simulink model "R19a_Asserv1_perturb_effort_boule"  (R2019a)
settings: Solver=ode15s  StartTime=0.0  StopTime=1  RelTol=1e-3  EnableMultiTasking=on
undefined symbols (not defined in the file): deg, kg, m, manette1_Défaut_sldprt, manette2_Défaut_sldprt, mm, N, rad, s, sigbuilder_block, STL, X, Y, Z
libraries: sm_lib x460, fl_lib x45, nesl_utility x23, simulink x3
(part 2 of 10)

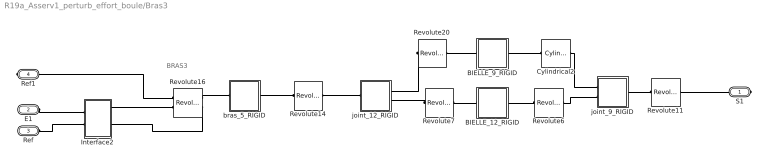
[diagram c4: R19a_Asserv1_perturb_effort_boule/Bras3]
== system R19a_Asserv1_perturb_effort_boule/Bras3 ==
  note: BRAS3
  BIELLE_12_RIGID : Subsystem
  BIELLE_9_RIGID : Subsystem
  Cylindrical2 : sm_lib/Joints/Cylindrical Joint  SenseConstraintForce=off  SenseConstraintForceX=off  SenseConstraintForceY=off  SenseConstraintForceZ=off  SenseConstraintTorque=off  SenseConstraintTorqueX=off  SenseConstraintTorqueY=off  SenseConstraintTorqueZ=off  SenseTotalForce=off  SenseTotalForceX=off  SenseTotalForceY=off  SenseTotalForceZ=off  SenseTotalTorque=off  SenseTotalTorqueX=off  SenseTotalTorqueY=off  SenseTotalTorqueZ=off  CompositeWrenchDir=FollowerOnBase  CompositeWrenchFrame=BaseFrame  PzEquilibriumPosition=0  PzEquilibriumPositionUnits=m  PzSpringStiffness=0  PzSpringStiffnessUnits=N/m  PzDampingCoefficient=0  PzDampingCoefficientUnits=s*N/m  PzTorqueActuationMode=NoTorque  PzMotionActuationMode=ComputedMotion  PzSensePosition=off  PzSenseVelocity=off  PzSenseAcceleration=off  PzSenseTorqueForce=off  PzSenseLowerLimitTorqueForce=off  PzSenseUpperLimitTorqueForce=off  PzLowerLimitSpecify=off  PzLowerLimitBound=-1  PzLowerLimitBoundUnits=m  PzLowerLimitStiffness=1e6  PzLowerLimitStiffnessUnits=N/m  PzLowerLimitDamping=1e3  PzLowerLimitDampingUnits=N/(m/s)  PzLowerLimitTransitionRegionWidth=1e-4  PzLowerLimitTransitionRegionWidthUnits=m  PzUpperLimitSpecify=off  PzUpperLimitBound=1  PzUpperLimitBoundUnits=m  PzUpperLimitStiffness=1e6  PzUpperLimitStiffnessUnits=N/m  PzUpperLimitDamping=1e3  PzUpperLimitDampingUnits=N/(m/s)  PzUpperLimitTransitionRegionWidth=1e-4  PzUpperLimitTransitionRegionWidthUnits=m  PzPositionTargetSpecify=off  PzPositionTargetPriority=High  PzPositionTargetValue=0  PzPositionTargetValueUnits=m  PzVelocityTargetSpecify=off  PzVelocityTargetPriority=High  PzVelocityTargetValue=0  PzVelocityTargetValueUnits=m/s  RzEquilibriumPosition=0  RzEquilibriumPositionUnits=rad  RzSpringStiffness=0  RzSpringStiffnessUnits=m*N/rad  RzDampingCoefficient=0  RzDampingCoefficientUnits=m*s*N/rad  RzTorqueActuationMode=NoTorque  RzMotionActuationMode=ComputedMotion  RzSensePosition=off  RzSenseVelocity=off  RzSenseAcceleration=off  RzSenseTorqueForce=off  RzSenseLowerLimitTorqueForce=off  RzSenseUpperLimitTorqueForce=off  RzLowerLimitSpecify=off  RzLowerLimitBound=-90  RzLowerLimitBoundUnits=deg  RzLowerLimitStiffness=1e4  RzLowerLimitStiffnessUnits=N*m/deg  RzLowerLimitDamping=10  RzLowerLimitDampingUnits=N*m/(deg/s)  RzLowerLimitTransitionRegionWidth=0.1  RzLowerLimitTransitionRegionWidthUnits=deg  RzUpperLimitSpecify=off  RzUpperLimitBound=90  RzUpperLimitBoundUnits=deg  RzUpperLimitStiffness=1e4  RzUpperLimitStiffnessUnits=N*m/deg  RzUpperLimitDamping=10  RzUpperLimitDampingUnits=N*m/(deg/s)  RzUpperLimitTransitionRegionWidth=0.1  RzUpperLimitTransitionRegionWidthUnits=deg  RzPositionTargetSpecify=off  RzPositionTargetPriority=High  RzPositionTargetValue=0  RzPositionTargetValueUnits=deg  RzVelocityTargetSpecify=off  RzVelocityTargetPriority=High  RzVelocityTargetValue=0  RzVelocityTargetValueUnits=deg/s
  Interface2 : Subsystem
  Revolute11 : sm_lib/Joints/Revolute Joint  SenseConstraintForce=off  SenseConstraintForceX=off  SenseConstraintForceY=off  SenseConstraintForceZ=off  SenseConstraintTorque=off  SenseConstraintTorqueX=off  SenseConstraintTorqueY=off  SenseConstraintTorqueZ=off  SenseTotalForce=off  SenseTotalForceX=off  SenseTotalForceY=off  SenseTotalForceZ=off  SenseTotalTorque=off  SenseTotalTorqueX=off  SenseTotalTorqueY=off  SenseTotalTorqueZ=off  CompositeWrenchDir=FollowerOnBase  CompositeWrenchFrame=BaseFrame  EquilibriumPosition=0  EquilibriumPositionUnits=rad  SpringStiffness=0  SpringStiffnessUnits=m*N/rad  DampingCoefficient=0  DampingCoefficientUnits=m*s*N/rad  TorqueActuationMode=NoTorque  MotionActuationMode=ComputedMotion  SensePosition=off  SenseVelocity=off  SenseAcceleration=off  SenseTorqueForce=off  SenseLowerLimitTorqueForce=off  SenseUpperLimitTorqueForce=off  LowerLimitSpecify=off  LowerLimitBound=-90  LowerLimitBoundUnits=deg  LowerLimitStiffness=1e4  LowerLimitStiffnessUnits=N*m/deg  LowerLimitDamping=10  LowerLimitDampingUnits=N*m/(deg/s)  LowerLimitTransitionRegionWidth=0.1  LowerLimitTransitionRegionWidthUnits=deg  UpperLimitSpecify=off  UpperLimitBound=90  UpperLimitBoundUnits=deg  UpperLimitStiffness=1e4  UpperLimitStiffnessUnits=N*m/deg  UpperLimitDamping=10  UpperLimitDampingUnits=N*m/(deg/s)  UpperLimitTransitionRegionWidth=0.1  UpperLimitTransitionRegionWidthUnits=deg  PositionTargetSpecify=on  PositionTargetPriority=Low  PositionTargetValue=36.757042846011267  PositionTargetValueUnits=deg  VelocityTargetSpecify=off  VelocityTargetPriority=High  VelocityTargetValue=0  VelocityTargetValueUnits=deg/s
  Revolute14 : sm_lib/Joints/Revolute Joint  SenseConstraintForce=off  SenseConstraintForceX=off  SenseConstraintForceY=off  SenseConstraintForceZ=off  SenseConstraintTorque=off  SenseConstraintTorqueX=off  SenseConstraintTorqueY=off  SenseConstraintTorqueZ=off  SenseTotalForce=off  SenseTotalForceX=off  SenseTotalForceY=off  SenseTotalForceZ=off  SenseTotalTorque=off  SenseTotalTorqueX=off  SenseTotalTorqueY=off  SenseTotalTorqueZ=off  CompositeWrenchDir=FollowerOnBase  CompositeWrenchFrame=BaseFrame  EquilibriumPosition=0  EquilibriumPositionUnits=rad  SpringStiffness=0  SpringStiffnessUnits=m*N/rad  DampingCoefficient=0  DampingCoefficientUnits=m*s*N/rad  TorqueActuationMode=NoTorque  MotionActuationMode=ComputedMotion  SensePosition=off  SenseVelocity=off  SenseAcceleration=off  SenseTorqueForce=off  SenseLowerLimitTorqueForce=off  SenseUpperLimitTorqueForce=off  LowerLimitSpecify=off  LowerLimitBound=-90  LowerLimitBoundUnits=deg  LowerLimitStiffness=1e4  LowerLimitStiffnessUnits=N*m/deg  LowerLimitDamping=10  LowerLimitDampingUnits=N*m/(deg/s)  LowerLimitTransitionRegionWidth=0.1  LowerLimitTransitionRegionWidthUnits=deg  UpperLimitSpecify=off  UpperLimitBound=90  UpperLimitBoundUnits=deg  UpperLimitStiffness=1e4  UpperLimitStiffnessUnits=N*m/deg  UpperLimitDamping=10  UpperLimitDampingUnits=N*m/(deg/s)  UpperLimitTransitionRegionWidth=0.1  UpperLimitTransitionRegionWidthUnits=deg  PositionTargetSpecify=on  PositionTargetPriority=Low  PositionTargetValue=114.86123956506862  PositionTargetValueUnits=deg  VelocityTargetSpecify=off  VelocityTargetPriority=High  VelocityTargetValue=0  VelocityTargetValueUnits=deg/s
  Revolute16 : sm_lib/Joints/Revolute Joint  SenseConstraintForce=off  SenseConstraintForceX=off  SenseConstraintForceY=off  SenseConstraintForceZ=off  SenseConstraintTorque=off  SenseConstraintTorqueX=off  SenseConstraintTorqueY=off  SenseConstraintTorqueZ=off  SenseTotalForce=off  SenseTotalForceX=off  SenseTotalForceY=off  SenseTotalForceZ=off  SenseTotalTorque=off  SenseTotalTorqueX=off  SenseTotalTorqueY=off  SenseTotalTorqueZ=off  CompositeWrenchDir=FollowerOnBase  CompositeWrenchFrame=BaseFrame  EquilibriumPosition=0  EquilibriumPositionUnits=rad  SpringStiffness=0  SpringStiffnessUnits=m*N/rad  DampingCoefficient=0  DampingCoefficientUnits=m*s*N/rad  TorqueActuationMode=InputTorque  MotionActuationMode=ComputedMotion  SensePosition=off  SenseVelocity=on  SenseAcceleration=off  SenseTorqueForce=off  SenseLowerLimitTorqueForce=off  SenseUpperLimitTorqueForce=off  LowerLimitSpecify=off  LowerLimitBound=-90  LowerLimitBoundUnits=deg  LowerLimitStiffness=1e4  LowerLimitStiffnessUnits=N*m/deg  LowerLimitDamping=10  LowerLimitDampingUnits=N*m/(deg/s)  LowerLimitTransitionRegionWidth=0.1  LowerLimitTransitionRegionWidthUnits=deg  UpperLimitSpecify=off  UpperLimitBound=90  UpperLimitBoundUnits=deg  UpperLimitStiffness=1e4  UpperLimitStiffnessUnits=N*m/deg  UpperLimitDamping=10  UpperLimitDampingUnits=N*m/(deg/s)  UpperLimitTransitionRegionWidth=0.1  UpperLimitTransitionRegionWidthUnits=deg  PositionTargetSpecify=on  PositionTargetPriority=Low  PositionTargetValue=101.89580328094226  PositionTargetValueUnits=deg  VelocityTargetSpecify=off  VelocityTargetPriority=High  VelocityTargetValue=0  VelocityTargetValueUnits=deg/s
  Revolute20 : sm_lib/Joints/Revolute Joint  SenseConstraintForce=off  SenseConstraintForceX=off  SenseConstraintForceY=off  SenseConstraintForceZ=off  SenseConstraintTorque=off  SenseConstraintTorqueX=off  SenseConstraintTorqueY=off  SenseConstraintTorqueZ=off  SenseTotalForce=off  SenseTotalForceX=off  SenseTotalForceY=off  SenseTotalForceZ=off  SenseTotalTorque=off  SenseTotalTorqueX=off  SenseTotalTorqueY=off  SenseTotalTorqueZ=off  CompositeWrenchDir=FollowerOnBase  CompositeWrenchFrame=BaseFrame  EquilibriumPosition=0  EquilibriumPositionUnits=rad  SpringStiffness=0  SpringStiffnessUnits=m*N/rad  DampingCoefficient=0  DampingCoefficientUnits=m*s*N/rad  TorqueActuationMode=NoTorque  MotionActuationMode=ComputedMotion  SensePosition=off  SenseVelocity=off  SenseAcceleration=off  SenseTorqueForce=off  SenseLowerLimitTorqueForce=off  SenseUpperLimitTorqueForce=off  LowerLimitSpecify=off  LowerLimitBound=-90  LowerLimitBoundUnits=deg  LowerLimitStiffness=1e4  LowerLimitStiffnessUnits=N*m/deg  LowerLimitDamping=10  LowerLimitDampingUnits=N*m/(deg/s)  LowerLimitTransitionRegionWidth=0.1  LowerLimitTransitionRegionWidthUnits=deg  UpperLimitSpecify=off  UpperLimitBound=90  UpperLimitBoundUnits=deg  UpperLimitStiffness=1e4  UpperLimitStiffnessUnits=N*m/deg  UpperLimitDamping=10  UpperLimitDampingUnits=N*m/(deg/s)  UpperLimitTransitionRegionWidth=0.1  UpperLimitTransitionRegionWidthUnits=deg  PositionTargetSpecify=on  PositionTargetPriority=Low  PositionTargetValue=-178.83470303505044  PositionTargetValueUnits=deg  VelocityTargetSpecify=off  VelocityTargetPriority=High  VelocityTargetValue=0  VelocityTargetValueUnits=deg/s
  Revolute6 : sm_lib/Joints/Revolute Joint  SenseConstraintForce=off  SenseConstraintForceX=off  SenseConstraintForceY=off  SenseConstraintForceZ=off  SenseConstraintTorque=off  SenseConstraintTorqueX=off  SenseConstraintTorqueY=off  SenseConstraintTorqueZ=off  SenseTotalForce=off  SenseTotalForceX=off  SenseTotalForceY=off  SenseTotalForceZ=off  SenseTotalTorque=off  SenseTotalTorqueX=off  SenseTotalTorqueY=off  SenseTotalTorqueZ=off  CompositeWrenchDir=FollowerOnBase  CompositeWrenchFrame=BaseFrame  EquilibriumPosition=0  EquilibriumPositionUnits=rad  SpringStiffness=0  SpringStiffnessUnits=m*N/rad  DampingCoefficient=0  DampingCoefficientUnits=m*s*N/rad  TorqueActuationMode=NoTorque  MotionActuationMode=ComputedMotion  SensePosition=off  SenseVelocity=off  SenseAcceleration=off  SenseTorqueForce=off  SenseLowerLimitTorqueForce=off  SenseUpperLimitTorqueForce=off  LowerLimitSpecify=off  LowerLimitBound=-90  LowerLimitBoundUnits=deg  LowerLimitStiffness=1e4  LowerLimitStiffnessUnits=N*m/deg  LowerLimitDamping=10  LowerLimitDampingUnits=N*m/(deg/s)  LowerLimitTransitionRegionWidth=0.1  LowerLimitTransitionRegionWidthUnits=deg  UpperLimitSpecify=off  UpperLimitBound=90  UpperLimitBoundUnits=deg  UpperLimitStiffness=1e4  UpperLimitStiffnessUnits=N*m/deg  UpperLimitDamping=10  UpperLimitDampingUnits=N*m/(deg/s)  UpperLimitTransitionRegionWidth=0.1  UpperLimitTransitionRegionWidthUnits=deg  PositionTargetSpecify=on  PositionTargetPriority=Low  PositionTargetValue=-178.83470303504936  PositionTargetValueUnits=deg  VelocityTargetSpecify=off  VelocityTargetPriority=High  VelocityTargetValue=0  VelocityTargetValueUnits=deg/s
  Revolute7 : sm_lib/Joints/Revolute Joint  SenseConstraintForce=off  SenseConstraintForceX=off  SenseConstraintForceY=off  SenseConstraintForceZ=off  SenseConstraintTorque=off  SenseConstraintTorqueX=off  SenseConstraintTorqueY=off  SenseConstraintTorqueZ=off  SenseTotalForce=off  SenseTotalForceX=off  SenseTotalForceY=off  SenseTotalForceZ=off  SenseTotalTorque=off  SenseTotalTorqueX=off  SenseTotalTorqueY=off  SenseTotalTorqueZ=off  CompositeWrenchDir=FollowerOnBase  CompositeWrenchFrame=BaseFrame  EquilibriumPosition=0  EquilibriumPositionUnits=rad  SpringStiffness=0  SpringStiffnessUnits=m*N/rad  DampingCoefficient=0  DampingCoefficientUnits=m*s*N/rad  TorqueActuationMode=NoTorque  MotionActuationMode=ComputedMotion  SensePosition=off  SenseVelocity=off  SenseAcceleration=off  SenseTorqueForce=off  SenseLowerLimitTorqueForce=off  SenseUpperLimitTorqueForce=off  LowerLimitSpecify=off  LowerLimitBound=-90  LowerLimitBoundUnits=deg  LowerLimitStiffness=1e4  LowerLimitStiffnessUnits=N*m/deg  LowerLimitDamping=10  LowerLimitDampingUnits=N*m/(deg/s)  LowerLimitTransitionRegionWidth=0.1  LowerLimitTransitionRegionWidthUnits=deg  UpperLimitSpecify=off  UpperLimitBound=90  UpperLimitBoundUnits=deg  UpperLimitStiffness=1e4  UpperLimitStiffnessUnits=N*m/deg  UpperLimitDamping=10  UpperLimitDampingUnits=N*m/(deg/s)  UpperLimitTransitionRegionWidth=0.1  UpperLimitTransitionRegionWidthUnits=deg  PositionTargetSpecify=on  PositionTargetPriority=Low  PositionTargetValue=1.1652969649496245  PositionTargetValueUnits=deg  VelocityTargetSpecify=off  VelocityTargetPriority=High  VelocityTargetValue=0  VelocityTargetValueUnits=deg/s
  bras_5_RIGID : Subsystem
  joint_12_RIGID : Subsystem
  joint_9_RIGID : Subsystem
  S1 : PMIOPort  Side=Right
  E1 : PMIOPort  Port=2  Side=Left
  Ref : PMIOPort  Port=3  Side=Left
  Ref1 : PMIOPort  Port=4  Side=Right
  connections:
  Interface2/RConn2 -- Revolute16/RConn2
  Interface2/RConn1 -- Revolute16/LConn2
  E1/RConn1 -- Interface2/LConn1
  Ref/RConn1 -- Interface2/LConn2
  Revolute11/RConn1 -- joint_9_RIGID/RConn1
  Revolute7/RConn1 -- joint_12_RIGID/RConn2
  Revolute14/RConn1 -- joint_12_RIGID/LConn1
  S1/RConn1 -- Revolute11/LConn1
  Revolute14/LConn1 -- bras_5_RIGID/RConn1
  Revolute16/LConn1 -- Ref1/RConn1
  Revolute16/RConn1 -- bras_5_RIGID/LConn1
  BIELLE_12_RIGID/RConn1 -- Revolute6/LConn1
  BIELLE_12_RIGID/LConn1 -- Revolute7/LConn1
  Revolute6/RConn1 -- joint_9_RIGID/LConn2
  Revolute20/RConn1 -- joint_12_RIGID/RConn1
  BIELLE_9_RIGID/LConn1 -- Revolute20/LConn1
  BIELLE_9_RIGID/RConn1 -- Cylindrical2/LConn1
  Cylindrical2/RConn1 -- joint_9_RIGID/LConn1

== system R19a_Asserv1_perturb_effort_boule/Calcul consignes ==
  note: a = 0.06; b = 0.1025; c = 0.014; d = 0.01125; e = 0.01125; f = 0.025 ; r = 0.03723; s = 0.02733;
  In1 : Inport
  In2 : Inport  Port=2
  In3 : Inport  Port=3
  AngleMoteur1 : MATLAB Function  TreatAsAtomicUnit=on
  AngleMoteur2 : MATLAB Function  TreatAsAtomicUnit=on
  AngleMoteur3 : MATLAB Function  TreatAsAtomicUnit=on
  C1 : Outport
  C2 : Outport  Port=2
  C3 : Outport  Port=3
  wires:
  In3/1 -> AngleMoteur1/3(z), AngleMoteur2/3(z), AngleMoteur3/3(z)
  AngleMoteur2/1(anglmot2) -> C2/1  "Consigne2"
  In1/1 -> AngleMoteur1/1(x), AngleMoteur2/1(x), AngleMoteur3/1(x)
  In2/1 -> AngleMoteur1/2(y), AngleMoteur2/2(y), AngleMoteur3/2(y)
  AngleMoteur1/1(anglmot1) -> C1/1  "Consigne1"
  AngleMoteur3/1(anglmot3) -> C3/1  "Consigne3"

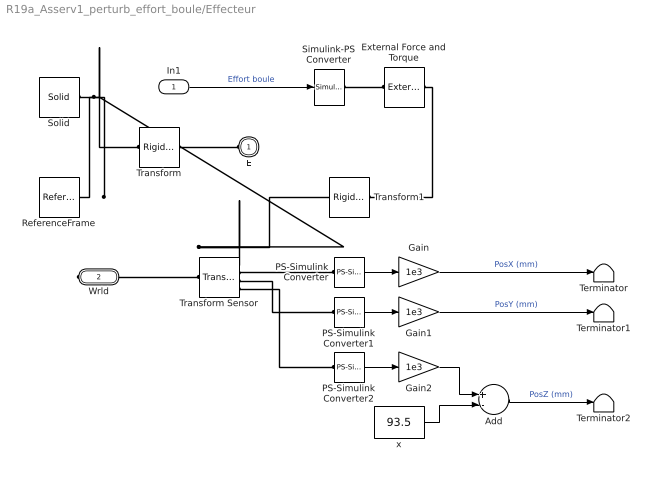
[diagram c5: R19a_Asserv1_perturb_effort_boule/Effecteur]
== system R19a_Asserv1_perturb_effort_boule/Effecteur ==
  In1 : Inport
  Add : Sum  Inputs=+-
  External Force and Torque : sm_lib/Forces and Torques/External Force and Torque  ForceResolutionFrame=AttachedFrame  EnableForceX=off  EnableForceY=off  EnableForceZ=on  EnableForce=off  TorqueResolutionFrame=AttachedFrame  EnableTorqueX=off  EnableTorqueY=off  EnableTorqueZ=off  EnableTorque=off
  Gain : Gain  Gain=1e3
  Gain1 : Gain  Gain=1e3
  Gain2 : Gain  Gain=1e3
  PS-Simulink Converter : nesl_utility/PS-Simulink Converter  PhysicalDomain=network_engine_domain  SubClassName=ps_output  LeftPortType=input  RightPortType=output  PseudoPeriodic=off  Frequencies=[]  Unit=1  AffineConversion=off
  PS-Simulink Converter1 : nesl_utility/PS-Simulink Converter  PhysicalDomain=network_engine_domain  SubClassName=ps_output  LeftPortType=input  RightPortType=output  PseudoPeriodic=off  Frequencies=[]  Unit=1  AffineConversion=off
  PS-Simulink Converter2 : nesl_utility/PS-Simulink Converter  PhysicalDomain=network_engine_domain  SubClassName=ps_output  LeftPortType=input  RightPortType=output  PseudoPeriodic=off  Frequencies=[]  Unit=1  AffineConversion=off
  ReferenceFrame : sm_lib/Frames and Transforms/Reference Frame
  Simulink-PS Converter : nesl_utility/Simulink-PS Converter  PhysicalDomain=network_engine_domain  SubClassName=ps_input  LeftPortType=input  RightPortType=output  PseudoPeriodic=off  Frequencies=[]  NoiseDistribution=none  NoiseParameters=[]  Unit=1  AffineConversion=off  FilteringAndDerivatives=zero  SimscapeFilterOrder=1  InputFilterTimeConstant=0.001  UdotUserProvided=1
  Solid : sm_lib/Body Elements/Solid  InertiaType=Custom  Mass=0.053  MassUnits=kg  CenterOfMass=[0 0 35.7]  CenterOfMassUnits=mm  MomentsOfInertia=[11.53195593564609 11.464562757624146 11.477456236480506]  MomentsOfInertiaUnits=kg*mm^2  ProductsOfInertia=[-0.014032469477280249 0.0038968914795150661 0.025527028661124163]  ProductsOfInertiaUnits=kg*mm^2  BasedOnType=Density  Density=1000  DensityUnits=kg/(m^3)  DoExposeReferenceFrame=on  SerializedFrames=<Frames/>  GraphicType=FromGeometry  MarkerShape=Sphere  MarkerSize=10  MarkerSizeUnits=m  GraphicVisPropType=SimpleVisualProperties  GraphicDiffuseColor=[1 1 1]  GraphicSpecularColor=[0.5 0.5 0.5 1.0]  GraphicAmbientColor=[0.15 0.15 0.15 1.0]  GraphicEmissiveColor=[0.0 0.0 0.0 1.0]  GraphicShininess=75  GraphicOpacity=1  GeometryShape=FromFile  RectangleSize=[1 1]  RectangleSizeUnits=m  BrickDimensions=[1 1 1]  BrickDimensionUnits=m  CylinderRadius=1  CylinderRadiusUnits=m  CylinderLength=1  CylinderLengthUnits=m  SphereRadius=1  SphereRadiusUnits=m  EllipsoidRadii=[1 1 1]  EllipsoidRadiiUnits=m  ExtrusionCrossSection=[1 1; -1 1; -1 -1; 1 -1]  ExtrusionCrossSectionUnits=m  ExtrusionLength=1  ExtrusionLengthUnits=m  PolygonNumSides=3  PolygonOuterRadius=1  PolygonOuterRadiusUnits=m  ExtGeomFileType=STL  ExtGeomFileName=\STL\manette2_Défaut_sldprt.STL  ExtGeomFileUnits=mm  RevolutionCrossSection=[1 1; 1 -1; 2 -1; 2 1]  RevolutionCrossSectionUnits=m  RevolutionExtent=Full  RevolutionAngle=180  RevolutionAngleUnits=deg
  Terminator : Terminator
  Terminator1 : Terminator
  Terminator2 : Terminator
  Transform : sm_lib/Frames and Transforms/Rigid Transform  TranslationMethod=Cartesian  TranslationStandardOffset=0  TranslationLengthUnit=mm  TranslationStandardAxis=+Z  TranslationCartesianOffset=[-0.52204305767083048 1.5422448888264837 -2.2456176397956377e-14]  TranslationROffset=0  TranslationROffsetUnits=m  TranslationZOffset=0  TranslationZOffsetUnits=m  TranslationThetaOffset=0  TranslationThetaOffsetUnits=deg  RotationMethod=ArbitraryAxis  RotationAngleUnits=rad  RotationStandardAxis=+Z  RotationAngle=2.2920311904365782  RotationArbitraryAxis=[0.63063758405056181 -0.45231899713116352 0.63063758405056158]  FollAlignAxisA=+X  BaseAlignAxisA=+Y  FollAlignAxisB=+Y  BaseAlignAxisB=+Z  RotationSequenceAxes=FollowerAxes  RotationSequence=XYX  RotationSequenceAngles=[0 0 0]  RotationSequenceAnglesUnits=deg  RotationMatrix=[1 0 0; 0 1 0; 0 0 1]
  Transform Sensor : sm_lib/Frames and Transforms/Transform Sensor  MeasurementFrame=World  SenseAngle=off  SenseAxis=off  SenseAngle1=off  SenseAngle2=off  SenseAngle3=off  SenseQ=off  SenseR=off  SenseOmegaX=off  SenseOmegaY=off  SenseOmegaZ=off  SenseOmega1=off  SenseOmega2=off  SenseOmega3=off  SenseQDot=off  SenseRDot=off  SenseAlphaX=off  SenseAlphaY=off  SenseAlphaZ=off  SenseAlpha1=off  SenseAlpha2=off  SenseAlpha3=off  SenseQDDot=off  SenseRDDot=off  SenseX=on  SenseY=on  SenseZ=on  SenseRad=off  SenseAzim=off  SenseDist=off  SenseInc=off  SenseXDot=off  SenseYDot=off  SenseZDot=off  SenseRadDot=off  SenseAzimDot=off  SenseDistDot=off  SenseIncDot=off  SenseXDDot=off  SenseYDDot=off  SenseZDDot=off  SenseRadDDot=off  SenseAzimDDot=off  SenseDistDDot=off  SenseIncDDot=off
  Transform1 : sm_lib/Frames and Transforms/Rigid Transform  TranslationMethod=None  TranslationStandardOffset=3  TranslationLengthUnit=mm  TranslationStandardAxis=-Z  TranslationCartesianOffset=[0 0 0]  TranslationROffset=0  TranslationROffsetUnits=m  TranslationZOffset=0  TranslationZOffsetUnits=m  TranslationThetaOffset=0  TranslationThetaOffsetUnits=deg  RotationMethod=None  RotationAngleUnits=rad  RotationStandardAxis=+Z  RotationAngle=2.2920311904365782  RotationArbitraryAxis=[0 0 0]  FollAlignAxisA=+X  BaseAlignAxisA=+Y  FollAlignAxisB=+Y  BaseAlignAxisB=+Z  RotationSequenceAxes=FollowerAxes  RotationSequence=XYX  RotationSequenceAngles=[0 0 0]  RotationSequenceAnglesUnits=deg  RotationMatrix=[1 0 0; 0 1 0; 0 0 1]
  x : Constant  Value=93.5
  E : PMIOPort  Side=Left
  Wrld : PMIOPort  Port=2  Side=Right
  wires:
  Gain1/1 -> Terminator1/1  "PosY (mm)"
  PS-Simulink Converter2/1 -> Gain2/1
  x/1 -> Add/2
  Add/1 -> Terminator2/1  "PosZ (mm)"
  PS-Simulink Converter1/1 -> Gain1/1
  Gain2/1 -> Add/1
  PS-Simulink Converter/1 -> Gain/1
  Gain/1 -> Terminator/1  "PosX (mm)"
  In1/1 -> Simulink-PS Converter/1  "Effort boule"
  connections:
  Solid/RConn1 -- ReferenceFrame/RConn1 -- Transform Sensor/RConn1 -- Transform1/RConn1 -- Transform/LConn1
  Transform/RConn1 -- E/RConn1
  Transform Sensor/RConn3 -- PS-Simulink Converter1/LConn1
  Wrld/RConn1 -- Transform Sensor/LConn1
  PS-Simulink Converter2/LConn1 -- Transform Sensor/RConn4
  Transform Sensor/RConn2 -- PS-Simulink Converter/LConn1
  Simulink-PS Converter/RConn1 -- External Force and Torque/LConn1
  External Force and Torque/RConn1 -- Transform1/LConn1

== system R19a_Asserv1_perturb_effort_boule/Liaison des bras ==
  EFFECTEUR_1_RIGID : Subsystem
  manette_1_RIGID : Subsystem
  E1 : PMIOPort  Side=Left
  E2 : PMIOPort  Port=2  Side=Left
  S1 : PMIOPort  Port=3  Side=Right
  E3 : PMIOPort  Port=4  Side=Left
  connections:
  EFFECTEUR_1_RIGID/RConn1 -- manette_1_RIGID/LConn1
  S1/RConn1 -- manette_1_RIGID/RConn1
  EFFECTEUR_1_RIGID/LConn1 -- E2/RConn1
  EFFECTEUR_1_RIGID/LConn3 -- E1/RConn1
  EFFECTEUR_1_RIGID/LConn2 -- E3/RConn1

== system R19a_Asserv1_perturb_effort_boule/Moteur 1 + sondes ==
  In1 : Inport
  Moteur à courant continu1 : Subsystem
  Reference electrique : fl_lib/Electrical/Electrical Elements/Electrical Reference
  Simulink-PS Converter1 : nesl_utility/Simulink-PS Converter  PhysicalDomain=network_engine_domain  SubClassName=ps_input  LeftPortType=input  RightPortType=output  PseudoPeriodic=off  Frequencies=[]  NoiseDistribution=none  NoiseParameters=[]  Unit=V  AffineConversion=off  FilteringAndDerivatives=zero  SimscapeFilterOrder=2  InputFilterTimeConstant=1e-4  UdotUserProvided=1
  Sondes électriques1 : Subsystem
  Source de tension controlée1 : fl_lib/Electrical/Electrical Sources/Controlled Voltage Source
  Conn1 : PMIOPort  Side=Right
  Conn2 : PMIOPort  Port=2  Side=Right
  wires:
  In1/1 -> Simulink-PS Converter1/1
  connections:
  Conn2/RConn1 -- Moteur à courant continu1/RConn2
  Conn1/RConn1 -- Moteur à courant continu1/RConn1
  Source de tension controlée1/LConn1 -- Sondes électriques1/LConn1
  Simulink-PS Converter1/RConn1 -- Source de tension controlée1/RConn1
  Sondes électriques1/RConn2 -- Source de tension controlée1/RConn2 -- Reference electrique/LConn1 -- Moteur à courant continu1/LConn2
  Sondes électriques1/RConn1 -- Moteur à courant continu1/LConn1

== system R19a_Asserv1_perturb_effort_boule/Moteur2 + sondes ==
  In1 : Inport
  Moteur à courant continu2 : Subsystem
  Reference electrique : fl_lib/Electrical/Electrical Elements/Electrical Reference
  Simulink-PS Converter1 : nesl_utility/Simulink-PS Converter  PhysicalDomain=network_engine_domain  SubClassName=ps_input  LeftPortType=input  RightPortType=output  PseudoPeriodic=off  Frequencies=[]  NoiseDistribution=none  NoiseParameters=[]  Unit=V  AffineConversion=off  FilteringAndDerivatives=zero  SimscapeFilterOrder=2  InputFilterTimeConstant=1e-4  UdotUserProvided=1
  Sondes électriques : Subsystem
  Source de tension controlée : fl_lib/Electrical/Electrical Sources/Controlled Voltage Source
  Conn1 : PMIOPort  Side=Right
  Conn2 : PMIOPort  Port=2  Side=Right
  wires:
  In1/1 -> Simulink-PS Converter1/1
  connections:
  Sondes électriques/RConn1 -- Moteur à courant continu2/LConn1
  Source de tension controlée/RConn2 -- Reference electrique/LConn1 -- Sondes électriques/RConn2 -- Moteur à courant continu2/LConn2
  Simulink-PS Converter1/RConn1 -- Source de tension controlée/RConn1
  Source de tension controlée/LConn1 -- Sondes électriques/LConn1
  Conn1/RConn1 -- Moteur à courant continu2/RConn1
  Conn2/RConn1 -- Moteur à courant continu2/RConn2

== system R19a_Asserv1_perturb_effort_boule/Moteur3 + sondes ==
  In1 : Inport
  Moteur à courant continu3 : Subsystem
  Reference electrique : fl_lib/Electrical/Electrical Elements/Electrical Reference
  Simulink-PS Converter1 : nesl_utility/Simulink-PS Converter  PhysicalDomain=network_engine_domain  SubClassName=ps_input  LeftPortType=input  RightPortType=output  PseudoPeriodic=off  Frequencies=[]  NoiseDistribution=none  NoiseParameters=[]  Unit=V  AffineConversion=off  FilteringAndDerivatives=zero  SimscapeFilterOrder=2  InputFilterTimeConstant=1e-4  UdotUserProvided=1
  Sondes électriques3 : Subsystem
  Source de tension controlée3 : fl_lib/Electrical/Electrical Sources/Controlled Voltage Source
  Conn1 : PMIOPort  Side=Right
  Conn2 : PMIOPort  Port=2  Side=Right
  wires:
  In1/1 -> Simulink-PS Converter1/1
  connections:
  Sondes électriques3/RConn1 -- Moteur à courant continu3/LConn1
  Moteur à courant continu3/LConn2 -- Reference electrique/LConn1 -- Source de tension controlée3/RConn2 -- Sondes électriques3/RConn2
  Simulink-PS Converter1/RConn1 -- Source de tension controlée3/RConn1
  Source de tension controlée3/LConn1 -- Sondes électriques3/LConn1
  Conn1/RConn1 -- Moteur à courant continu3/RConn1
  Conn2/RConn1 -- Moteur à courant continu3/RConn2

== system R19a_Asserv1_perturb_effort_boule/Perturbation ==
  Générateur de perturbation : Subsystem  Tag=STV Subsys  LoadFcn=sigbuilder_block('load');  StartFcn=sigbuilder_block('start');  StopFcn=sigbuilder_block('stop');  ClipboardFcn=sigbuilder_block('clipboard');  mask(Sigbuilder block){tuvar=[0:10]}
      mask help: Simulink:masks:SigbuilderBlock_MD
      mask init:
      | if ~strcmp(get_param(bdroot(gcbh),'SimulationStatus'),'stopped') tuvar = sigbuilder_block('maskInit'); end
  Nul : Constant  Value=0
  Out1 : Outport
  Out2 : Outport  Port=2
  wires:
  Générateur de perturbation/1(Signal 1) -> Out1/1  "On"
  Nul/1 -> Out2/1  "Off"

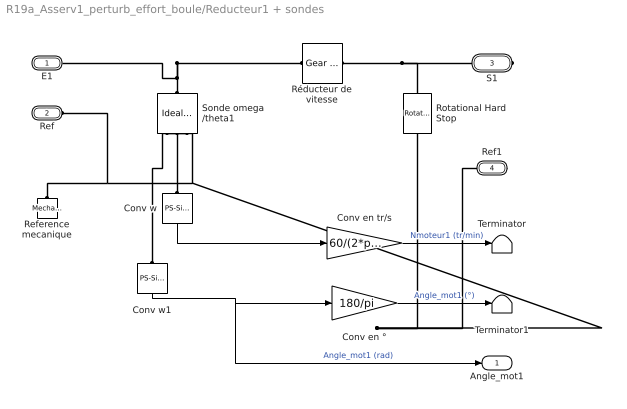
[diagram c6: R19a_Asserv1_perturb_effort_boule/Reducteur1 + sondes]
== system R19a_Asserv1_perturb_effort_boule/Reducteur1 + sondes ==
  Conv en tr/s : Gain  Gain=60/(2*pi)
  Conv en ° : Gain  Gain=180/pi
  Conv w : nesl_utility/PS-Simulink Converter  PhysicalDomain=network_engine_domain  SubClassName=ps_output  LeftPortType=input  RightPortType=output  PseudoPeriodic=off  Frequencies=[]  Unit=1  AffineConversion=off
  Conv w1 : nesl_utility/PS-Simulink Converter  PhysicalDomain=network_engine_domain  SubClassName=ps_output  LeftPortType=input  RightPortType=output  PseudoPeriodic=off  Frequencies=[]  Unit=1  AffineConversion=off
  Reference mecanique : fl_lib/Mechanical/Rotational Elements/Mechanical Rotational Reference
  Rotational Hard Stop : fl_lib/Mechanical/Rotational Elements/Rotational Hard Stop  upper_bnd=0 rad  lower_bnd=-2 rad  stiff_up=1e2 N*m/rad  stiff_low=1e2 N*m/rad  D_up=0.01 N*m/(rad/s)  D_low=0.01 N*m/(rad/s)  model=simscape.enum.hardstop.fulldamped  transition=0.001 rad  w_specify=off  w_priority=High  w=0 rad/s  w_nominal_specify=off  w_nominal_unit=rad/s  w_nominal_value=1  t_specify=off  t_priority=High  t=0 N*m  t_nominal_specify=off  t_nominal_unit=N*m  t_nominal_value=1  phi_specify=off  phi_priority=High  phi=0 rad  phi_nominal_specify=off  phi_nominal_unit=rad  phi_nominal_value=1
  Réducteur de vitesse : fl_lib/Mechanical/Mechanisms/Gear Box  ratio=-7.627  t_in_specify=off  t_in_priority=High  t_in=0 N*m  t_in_nominal_specify=off  t_in_nominal_unit=N*m  t_in_nominal_value=1  t_out_specify=off  t_out_priority=High  t_out=0 N*m  t_out_nominal_specify=off  t_out_nominal_unit=N*m  t_out_nominal_value=1
  Sonde omega /theta1 : fl_lib/Mechanical/Mechanical Sensors/Ideal Rotational Motion Sensor  offset=0 rad
  Terminator : Terminator
  Terminator1 : Terminator
  E1 : PMIOPort  Side=Left
  Ref : PMIOPort  Port=2  Side=Left
  S1 : PMIOPort  Port=3  Side=Right
  Ref1 : PMIOPort  Port=4  Side=Right
  Angle_mot1 : Outport
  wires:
  Conv w1/1 -> Angle_mot1/1, Conv en °/1  "Angle_mot1 (rad)"
  Conv en °/1 -> Terminator1/1  "Angle_mot1 (°)"
  Conv w/1 -> Conv en tr/s/1
  Conv en tr/s/1 -> Terminator/1  "Nmoteur1 (tr/min)"
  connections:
  Sonde omega /theta1/LConn1 -- E1/RConn1 -- Réducteur de vitesse/LConn1
  Reference mecanique/LConn1 -- Ref/RConn1 -- Rotational Hard Stop/RConn1 -- Ref1/RConn1 -- Sonde omega /theta1/RConn1
  Conv w/LConn1 -- Sonde omega /theta1/RConn2
  Conv w1/LConn1 -- Sonde omega /theta1/RConn3
  Réducteur de vitesse/RConn1 -- Rotational Hard Stop/LConn1 -- S1/RConn1

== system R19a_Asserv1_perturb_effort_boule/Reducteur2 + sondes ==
  Conv en tr/s : Gain  Gain=60/(2*pi)
  Conv en ° : Gain  Gain=180/pi
  Conv w : nesl_utility/PS-Simulink Converter  PhysicalDomain=network_engine_domain  SubClassName=ps_output  LeftPortType=input  RightPortType=output  PseudoPeriodic=off  Frequencies=[]  Unit=1  AffineConversion=off
  Conv w1 : nesl_utility/PS-Simulink Converter  PhysicalDomain=network_engine_domain  SubClassName=ps_output  LeftPortType=input  RightPortType=output  PseudoPeriodic=off  Frequencies=[]  Unit=1  AffineConversion=off
  Reference mecanique : fl_lib/Mechanical/Rotational Elements/Mechanical Rotational Reference
  Rotational Hard Stop : fl_lib/Mechanical/Rotational Elements/Rotational Hard Stop  upper_bnd=2 rad  lower_bnd=0 rad  stiff_up=1e2 N*m/rad  stiff_low=1e2 N*m/rad  D_up=0.01 N*m/(rad/s)  D_low=0.01 N*m/(rad/s)  model=simscape.enum.hardstop.fulldamped  transition=0.001 rad  w_specify=off  w_priority=High  w=0 rad/s  w_nominal_specify=off  w_nominal_unit=rad/s  w_nominal_value=1  t_specify=off  t_priority=High  t=0 N*m  t_nominal_specify=off  t_nominal_unit=N*m  t_nominal_value=1  phi_specify=off  phi_priority=High  phi=0 rad  phi_nominal_specify=off  phi_nominal_unit=rad  phi_nominal_value=1
  Réducteur de vitesse2 : fl_lib/Mechanical/Mechanisms/Gear Box  ratio=7.627  t_in_specify=off  t_in_priority=High  t_in=0 N*m  t_in_nominal_specify=off  t_in_nominal_unit=N*m  t_in_nominal_value=1  t_out_specify=off  t_out_priority=High  t_out=0 N*m  t_out_nominal_specify=off  t_out_nominal_unit=N*m  t_out_nominal_value=1
  Sonde omega /theta2 : fl_lib/Mechanical/Mechanical Sensors/Ideal Rotational Motion Sensor  offset=0 rad
  Terminator : Terminator
  Terminator1 : Terminator
  E1 : PMIOPort  Side=Left
  Ref : PMIOPort  Port=2  Side=Left
  S1 : PMIOPort  Port=3  Side=Right
  Ref1 : PMIOPort  Port=4  Side=Right
  Angle_mot2 : Outport
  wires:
  Conv w1/1 -> Angle_mot2/1, Conv en °/1  "Angle_mot2 (rad)"
  Conv en °/1 -> Terminator1/1  "Angle_mot2 (°)"
  Conv w/1 -> Conv en tr/s/1
  Conv en tr/s/1 -> Terminator/1  "Nmoteur2 (tr/min)"
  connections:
  Sonde omega /theta2/LConn1 -- E1/RConn1 -- Réducteur de vitesse2/LConn1
  Ref1/RConn1 -- Rotational Hard Stop/RConn1 -- Sonde omega /theta2/RConn1 -- Reference mecanique/LConn1 -- Ref/RConn1
  Conv w1/LConn1 -- Sonde omega /theta2/RConn3
  Conv w/LConn1 -- Sonde omega /theta2/RConn2
  Réducteur de vitesse2/RConn1 -- Rotational Hard Stop/LConn1 -- S1/RConn1

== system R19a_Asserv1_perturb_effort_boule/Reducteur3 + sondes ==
  Conv en tr/s : Gain  Gain=60/(2*pi)
  Conv en ° : Gain  Gain=180/pi
  Conv w : nesl_utility/PS-Simulink Converter  PhysicalDomain=network_engine_domain  SubClassName=ps_output  LeftPortType=input  RightPortType=output  PseudoPeriodic=off  Frequencies=[]  Unit=1  AffineConversion=off
  Conv w1 : nesl_utility/PS-Simulink Converter  PhysicalDomain=network_engine_domain  SubClassName=ps_output  LeftPortType=input  RightPortType=output  PseudoPeriodic=off  Frequencies=[]  Unit=1  AffineConversion=off
  Reference mecanique : fl_lib/Mechanical/Rotational Elements/Mechanical Rotational Reference
  Rotational Hard Stop : fl_lib/Mechanical/Rotational Elements/Rotational Hard Stop  upper_bnd=2 rad  lower_bnd=0 rad  stiff_up=1e2 N*m/rad  stiff_low=1e2 N*m/rad  D_up=0.01 N*m/(rad/s)  D_low=0.01 N*m/(rad/s)  model=simscape.enum.hardstop.fulldamped  transition=0.001 rad  w_specify=off  w_priority=High  w=0 rad/s  w_nominal_specify=off  w_nominal_unit=rad/s  w_nominal_value=1  t_specify=off  t_priority=High  t=0 N*m  t_nominal_specify=off  t_nominal_unit=N*m  t_nominal_value=1  phi_specify=off  phi_priority=High  phi=0 rad  phi_nominal_specify=off  phi_nominal_unit=rad  phi_nominal_value=1
  Réducteur de vitesse3 : fl_lib/Mechanical/Mechanisms/Gear Box  ratio=7.627  t_in_specify=off  t_in_priority=High  t_in=0 N*m  t_in_nominal_specify=off  t_in_nominal_unit=N*m  t_in_nominal_value=1  t_out_specify=off  t_out_priority=High  t_out=0 N*m  t_out_nominal_specify=off  t_out_nominal_unit=N*m  t_out_nominal_value=1
  Sonde omega /theta2 : fl_lib/Mechanical/Mechanical Sensors/Ideal Rotational Motion Sensor  offset=0 rad
  Terminator : Terminator
  Terminator1 : Terminator
  E1 : PMIOPort  Side=Left
  Ref : PMIOPort  Port=2  Side=Left
  S1 : PMIOPort  Port=3  Side=Right
  Ref1 : PMIOPort  Port=4  Side=Right
  Angle_mot3 : Outport
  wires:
  Conv w1/1 -> Angle_mot3/1, Conv en °/1  "Angle_mot3 (rad)"
  Conv en °/1 -> Terminator1/1  "Angle_mot3 (°)"
  Conv w/1 -> Conv en tr/s/1
  Conv en tr/s/1 -> Terminator/1  "Nmoteur3 (tr/min)"
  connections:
  Sonde omega /theta2/LConn1 -- E1/RConn1 -- Réducteur de vitesse3/LConn1
  Ref/RConn1 -- Reference mecanique/LConn1 -- Rotational Hard Stop/RConn1 -- Ref1/RConn1 -- Sonde omega /theta2/RConn1
  Conv w1/LConn1 -- Sonde omega /theta2/RConn3
  Réducteur de vitesse3/RConn1 -- Rotational Hard Stop/LConn1 -- S1/RConn1
  Conv w/LConn1 -- Sonde omega /theta2/RConn2

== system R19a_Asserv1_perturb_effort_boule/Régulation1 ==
  In1 : Inport
  In2 : Inport  Port=2
  P : Inport  Port=3
  I : Inport  Port=4
  D : Inport  Port=5
  Add : Sum  Inputs=-+
  Constant : Constant  Value=900
  Correcteur PID : simulink/Continuous/PID Controller  Controller=PID  Form=Parallel  TimeDomain=Continuous-time  SampleTime=-1  IntegratorMethod=Forward Euler  FilterMethod=Forward Euler  ControllerParametersSource=external  P=20  I=30  D=4  UseFilter=on  N=900  TunerSelectOption=Transfer Function Based (PID Tuner App)  ZeroCross=off  InitialConditionSource=internal  InitialConditionForIntegrator=0  InitialConditionForFilter=0  DifferentiatorICPrevScaledInput=0  ExternalReset=none  TrackingMode=off  Kt=1  LimitOutput=on  UpperSaturationLimit=30  LowerSaturationLimit=-30  LinearizeAsGain=off  AntiWindupMode=clamping  Kb=0.01  POutMin=[]  POutMax=[]  IOutMin=[]  IOutMax=[]  DOutMin=[]  DOutMax=[]  NOutMin=[]  NOutMax=[]  SumOutMin=[]  SumOutMax=[]  SaturationOutMin=[]  SaturationOutMax=[]  PParamMin=[]  PParamMax=[]  IParamMin=[]  IParamMax=[]  DParamMin=[]  DParamMax=[]  NParamMin=[]  NParamMax=[]  KbParamMin=[]  KbParamMax=[]  KtParamMin=[]  KtParamMax=[]  KbOutMin=[]  KbOutMax=[]  KtOutMin=[]  KtOutMax=[]  IntegratorOutMin=[]  IntegratorOutMax=[]  FilterOutMin=[]  FilterOutMax=[]  SumI1OutMin=[]  SumI1OutMax=[]  SumI2OutMin=[]  SumI2OutMax=[]  SumI3OutMin=[]  SumI3OutMax=[]  SumI4OutMin=[]  SumI4OutMax=[]  SumDOutMin=[]  SumDOutMax=[]  DifferentiatorOutMin=[]  DifferentiatorOutMax=[]  FilterDiffOutCoefMin=[]  FilterDiffOutCoefMax=[]  ReciprocalOutMin=[]  ReciprocalOutMax=[]  SumDenOutMin=[]  SumDenOutMax=[]  SumNumOutMin=[]  SumNumOutMax=[]  DivideOutMin=[]  DivideOutMax=[]  IntegratorContinuousStateAttributes=''  IntegratorStateMustResolveToSignalObject=off  IntegratorRTWStateStorageClass=Auto  FilterContinuousStateAttributes=''  FilterStateMustResolveToSignalObject=off  FilterRTWStateStorageClass=Auto  ParallelPVariant=ExternalParameters  IdealPVariant=Disabled  IVariant=ExternalParameters  DVariant=ExternalParameters  IntegratorVariant=Continuous  SatVariant=Enabled  AWVariant=ContClampingParallel  PCopyVariant=Disabled  TRVariant=Disabled  FdbkBlocksVariant=Forward  IdealPFdbkVariant=Disabled  SatFdbkVariant=Disabled  DerivativeFilterVariant=ContFilter  NVariant=ExternalParameters  NCopyVariant=Disabled  FilterICVariant=InternalICsFilter  IntegratorICVariant=InternalICs  ExternalResetVariant=Disabled  TRSumVariant=Passthrough  SumFdbkVariant=Disabled  SumVariant=Sum_PID
  Out1 : Outport
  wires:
  In1/1 -> Add/1
  In2/1 -> Add/2
  Correcteur PID/1 -> Out1/1
  Add/1 -> Correcteur PID/1
  Constant/1 -> Correcteur PID/5
  P/1 -> Correcteur PID/2
  I/1 -> Correcteur PID/3
  D/1 -> Correcteur PID/4

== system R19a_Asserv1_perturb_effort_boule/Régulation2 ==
  In1 : Inport
  In2 : Inport  Port=2
  P : Inport  Port=3
  I : Inport  Port=4
  D : Inport  Port=5
  Add : Sum  Inputs=-+
  Constant : Constant  Value=900
  Correcteur PID : simulink/Continuous/PID Controller  Controller=PID  Form=Parallel  TimeDomain=Continuous-time  SampleTime=-1  IntegratorMethod=Forward Euler  FilterMethod=Forward Euler  ControllerParametersSource=external  P=20  I=30  D=4  UseFilter=on  N=900  TunerSelectOption=Transfer Function Based (PID Tuner App)  ZeroCross=off  InitialConditionSource=internal  InitialConditionForIntegrator=0  InitialConditionForFilter=0  DifferentiatorICPrevScaledInput=0  ExternalReset=none  TrackingMode=off  Kt=1  LimitOutput=on  UpperSaturationLimit=30  LowerSaturationLimit=-30  LinearizeAsGain=off  AntiWindupMode=clamping  Kb=1  POutMin=[]  POutMax=[]  IOutMin=[]  IOutMax=[]  DOutMin=[]  DOutMax=[]  NOutMin=[]  NOutMax=[]  SumOutMin=[]  SumOutMax=[]  SaturationOutMin=[]  SaturationOutMax=[]  PParamMin=[]  PParamMax=[]  IParamMin=[]  IParamMax=[]  DParamMin=[]  DParamMax=[]  NParamMin=[]  NParamMax=[]  KbParamMin=[]  KbParamMax=[]  KtParamMin=[]  KtParamMax=[]  KbOutMin=[]  KbOutMax=[]  KtOutMin=[]  KtOutMax=[]  IntegratorOutMin=[]  IntegratorOutMax=[]  FilterOutMin=[]  FilterOutMax=[]  SumI1OutMin=[]  SumI1OutMax=[]  SumI2OutMin=[]  SumI2OutMax=[]  SumI3OutMin=[]  SumI3OutMax=[]  SumI4OutMin=[]  SumI4OutMax=[]  SumDOutMin=[]  SumDOutMax=[]  DifferentiatorOutMin=[]  DifferentiatorOutMax=[]  FilterDiffOutCoefMin=[]  FilterDiffOutCoefMax=[]  ReciprocalOutMin=[]  ReciprocalOutMax=[]  SumDenOutMin=[]  SumDenOutMax=[]  SumNumOutMin=[]  SumNumOutMax=[]  DivideOutMin=[]  DivideOutMax=[]  IntegratorContinuousStateAttributes=''  IntegratorStateMustResolveToSignalObject=off  IntegratorRTWStateStorageClass=Auto  FilterContinuousStateAttributes=''  FilterStateMustResolveToSignalObject=off  FilterRTWStateStorageClass=Auto  ParallelPVariant=ExternalParameters  IdealPVariant=Disabled  IVariant=ExternalParameters  DVariant=ExternalParameters  IntegratorVariant=Continuous  SatVariant=Enabled  AWVariant=ContClampingParallel  PCopyVariant=Disabled  TRVariant=Disabled  FdbkBlocksVariant=Forward  IdealPFdbkVariant=Disabled  SatFdbkVariant=Disabled  DerivativeFilterVariant=ContFilter  NVariant=ExternalParameters  NCopyVariant=Disabled  FilterICVariant=InternalICsFilter  IntegratorICVariant=InternalICs  ExternalResetVariant=Disabled  TRSumVariant=Passthrough  SumFdbkVariant=Disabled  SumVariant=Sum_PID
  Out1 : Outport
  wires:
  D/1 -> Correcteur PID/4
  I/1 -> Correcteur PID/3
  P/1 -> Correcteur PID/2
  Constant/1 -> Correcteur PID/5
  Add/1 -> Correcteur PID/1
  Correcteur PID/1 -> Out1/1
  In2/1 -> Add/2
  In1/1 -> Add/1

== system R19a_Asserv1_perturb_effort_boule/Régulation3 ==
  In1 : Inport
  In2 : Inport  Port=2
  P : Inport  Port=3
  I : Inport  Port=4
  D : Inport  Port=5
  Add : Sum  Inputs=-+
  Constant : Constant  Value=900
  Correcteur PID : simulink/Continuous/PID Controller  Controller=PID  Form=Parallel  TimeDomain=Continuous-time  SampleTime=-1  IntegratorMethod=Forward Euler  FilterMethod=Forward Euler  ControllerParametersSource=external  P=20  I=30  D=4  UseFilter=on  N=900  TunerSelectOption=Transfer Function Based (PID Tuner App)  ZeroCross=off  InitialConditionSource=internal  InitialConditionForIntegrator=0  InitialConditionForFilter=0  DifferentiatorICPrevScaledInput=0  ExternalReset=none  TrackingMode=off  Kt=1  LimitOutput=on  UpperSaturationLimit=30  LowerSaturationLimit=-30  LinearizeAsGain=off  AntiWindupMode=clamping  Kb=1  POutMin=[]  POutMax=[]  IOutMin=[]  IOutMax=[]  DOutMin=[]  DOutMax=[]  NOutMin=[]  NOutMax=[]  SumOutMin=[]  SumOutMax=[]  SaturationOutMin=[]  SaturationOutMax=[]  PParamMin=[]  PParamMax=[]  IParamMin=[]  IParamMax=[]  DParamMin=[]  DParamMax=[]  NParamMin=[]  NParamMax=[]  KbParamMin=[]  KbParamMax=[]  KtParamMin=[]  KtParamMax=[]  KbOutMin=[]  KbOutMax=[]  KtOutMin=[]  KtOutMax=[]  IntegratorOutMin=[]  IntegratorOutMax=[]  FilterOutMin=[]  FilterOutMax=[]  SumI1OutMin=[]  SumI1OutMax=[]  SumI2OutMin=[]  SumI2OutMax=[]  SumI3OutMin=[]  SumI3OutMax=[]  SumI4OutMin=[]  SumI4OutMax=[]  SumDOutMin=[]  SumDOutMax=[]  DifferentiatorOutMin=[]  DifferentiatorOutMax=[]  FilterDiffOutCoefMin=[]  FilterDiffOutCoefMax=[]  ReciprocalOutMin=[]  ReciprocalOutMax=[]  SumDenOutMin=[]  SumDenOutMax=[]  SumNumOutMin=[]  SumNumOutMax=[]  DivideOutMin=[]  DivideOutMax=[]  IntegratorContinuousStateAttributes=''  IntegratorStateMustResolveToSignalObject=off  IntegratorRTWStateStorageClass=Auto  FilterContinuousStateAttributes=''  FilterStateMustResolveToSignalObject=off  FilterRTWStateStorageClass=Auto  ParallelPVariant=ExternalParameters  IdealPVariant=Disabled  IVariant=ExternalParameters  DVariant=ExternalParameters  IntegratorVariant=Continuous  SatVariant=Enabled  AWVariant=ContClampingParallel  PCopyVariant=Disabled  TRVariant=Disabled  FdbkBlocksVariant=Forward  IdealPFdbkVariant=Disabled  SatFdbkVariant=Disabled  DerivativeFilterVariant=ContFilter  NVariant=ExternalParameters  NCopyVariant=Disabled  FilterICVariant=InternalICsFilter  IntegratorICVariant=InternalICs  ExternalResetVariant=Disabled  TRSumVariant=Passthrough  SumFdbkVariant=Disabled  SumVariant=Sum_PID
  Out1 : Outport
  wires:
  In1/1 -> Add/1
  In2/1 -> Add/2
  Correcteur PID/1 -> Out1/1
  Add/1 -> Correcteur PID/1
  Constant/1 -> Correcteur PID/5
  P/1 -> Correcteur PID/2
  I/1 -> Correcteur PID/3
  D/1 -> Correcteur PID/4

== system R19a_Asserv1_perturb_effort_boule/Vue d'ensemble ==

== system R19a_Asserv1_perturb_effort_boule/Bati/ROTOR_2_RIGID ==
  CODEUR_1_RIGID : Subsystem
  ROTOR_1_RIGID : Subsystem
  ReferenceFrame : sm_lib/Frames and Transforms/Reference Frame
  Transform : sm_lib/Frames and Transforms/Rigid Transform  TranslationMethod=Cartesian  TranslationStandardOffset=0  TranslationLengthUnit=mm  TranslationStandardAxis=+Z  TranslationCartesianOffset=[30.900000000000009 0 -2.4868995751603507e-14]  TranslationROffset=0  TranslationROffsetUnits=m  TranslationZOffset=0  TranslationZOffsetUnits=m  TranslationThetaOffset=0  TranslationThetaOffsetUnits=deg  RotationMethod=ArbitraryAxis  RotationAngleUnits=rad  RotationStandardAxis=+Z  RotationAngle=2.0943951023931953  RotationArbitraryAxis=[0.57735026918962584 0.57735026918962562 0.57735026918962584]  FollAlignAxisA=+X  BaseAlignAxisA=+Y  FollAlignAxisB=+Y  BaseAlignAxisB=+Z  RotationSequenceAxes=FollowerAxes  RotationSequence=XYX  RotationSequenceAngles=[0 0 0]  RotationSequenceAnglesUnits=deg  RotationMatrix=[1 0 0; 0 1 0; 0 0 1]
  Transform1 : sm_lib/Frames and Transforms/Rigid Transform  TranslationMethod=Cartesian  TranslationStandardOffset=0  TranslationLengthUnit=mm  TranslationStandardAxis=+Z  TranslationCartesianOffset=[30.899999999999991 0 0]  TranslationROffset=0  TranslationROffsetUnits=m  TranslationZOffset=0  TranslationZOffsetUnits=m  TranslationThetaOffset=0  TranslationThetaOffsetUnits=deg  RotationMethod=ArbitraryAxis  RotationAngleUnits=rad  RotationStandardAxis=+Z  RotationAngle=1.9381695666920589  RotationArbitraryAxis=[0.51405666735189148 -0.51405666735189148 0.68665237602598705]  FollAlignAxisA=+X  BaseAlignAxisA=+Y  FollAlignAxisB=+Y  BaseAlignAxisB=+Z  RotationSequenceAxes=FollowerAxes  RotationSequence=XYX  RotationSequenceAngles=[0 0 0]  RotationSequenceAnglesUnits=deg  RotationMatrix=[1 0 0; 0 1 0; 0 0 1]
  Transform2 : sm_lib/Frames and Transforms/Rigid Transform  TranslationMethod=Cartesian  TranslationStandardOffset=0  TranslationLengthUnit=mm  TranslationStandardAxis=+Z  TranslationCartesianOffset=[-36.399999999999999 0 0]  TranslationROffset=0  TranslationROffsetUnits=m  TranslationZOffset=0  TranslationZOffsetUnits=m  TranslationThetaOffset=0  TranslationThetaOffsetUnits=deg  RotationMethod=ArbitraryAxis  RotationAngleUnits=rad  RotationStandardAxis=+Z  RotationAngle=1.624664356272121  RotationArbitraryAxis=[-0.22603347840136132 0.22603347840136129 0.94753244444903439]  FollAlignAxisA=+X  BaseAlignAxisA=+Y  FollAlignAxisB=+Y  BaseAlignAxisB=+Z  RotationSequenceAxes=FollowerAxes  RotationSequence=XYX  RotationSequenceAngles=[0 0 0]  RotationSequenceAnglesUnits=deg  RotationMatrix=[1 0 0; 0 1 0; 0 0 1]
  F : PMIOPort  Side=Left
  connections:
  ReferenceFrame/RConn1 -- Transform/LConn1 -- Transform1/LConn1 -- Transform2/LConn1
  Transform/RConn1 -- F/RConn1
  ROTOR_1_RIGID/LConn1 -- Transform1/RConn1
  CODEUR_1_RIGID/LConn1 -- Transform2/RConn1

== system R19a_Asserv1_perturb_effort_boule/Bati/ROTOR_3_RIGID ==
  CODEUR_1_RIGID : Subsystem
  ROTOR_1_RIGID : Subsystem
  ReferenceFrame : sm_lib/Frames and Transforms/Reference Frame
  Transform : sm_lib/Frames and Transforms/Rigid Transform  TranslationMethod=Cartesian  TranslationStandardOffset=0  TranslationLengthUnit=mm  TranslationStandardAxis=+Z  TranslationCartesianOffset=[30.899999999999984 -7.1054273576010019e-15 1.7763568394002505e-15]  TranslationROffset=0  TranslationROffsetUnits=m  TranslationZOffset=0  TranslationZOffsetUnits=m  TranslationThetaOffset=0  TranslationThetaOffsetUnits=deg  RotationMethod=ArbitraryAxis  RotationAngleUnits=rad  RotationStandardAxis=+Z  RotationAngle=2.0943951023931953  RotationArbitraryAxis=[0.57735026918962562 0.57735026918962584 0.57735026918962595]  FollAlignAxisA=+X  BaseAlignAxisA=+Y  FollAlignAxisB=+Y  BaseAlignAxisB=+Z  RotationSequenceAxes=FollowerAxes  RotationSequence=XYX  RotationSequenceAngles=[0 0 0]  RotationSequenceAnglesUnits=deg  RotationMatrix=[1 0 0; 0 1 0; 0 0 1]
  Transform1 : sm_lib/Frames and Transforms/Rigid Transform  TranslationMethod=Cartesian  TranslationStandardOffset=0  TranslationLengthUnit=mm  TranslationStandardAxis=+Z  TranslationCartesianOffset=[30.899999999999999 0 0]  TranslationROffset=0  TranslationROffsetUnits=m  TranslationZOffset=0  TranslationZOffsetUnits=m  TranslationThetaOffset=0  TranslationThetaOffsetUnits=deg  RotationMethod=ArbitraryAxis  RotationAngleUnits=rad  RotationStandardAxis=+Z  RotationAngle=1.9381695666920589  RotationArbitraryAxis=[0.51405666735189148 -0.51405666735189148 0.68665237602598705]  FollAlignAxisA=+X  BaseAlignAxisA=+Y  FollAlignAxisB=+Y  BaseAlignAxisB=+Z  RotationSequenceAxes=FollowerAxes  RotationSequence=XYX  RotationSequenceAngles=[0 0 0]  RotationSequenceAnglesUnits=deg  RotationMatrix=[1 0 0; 0 1 0; 0 0 1]
  Transform2 : sm_lib/Frames and Transforms/Rigid Transform  TranslationMethod=Cartesian  TranslationStandardOffset=0  TranslationLengthUnit=mm  TranslationStandardAxis=+Z  TranslationCartesianOffset=[-36.399999999999999 0 0]  TranslationROffset=0  TranslationROffsetUnits=m  TranslationZOffset=0  TranslationZOffsetUnits=m  TranslationThetaOffset=0  TranslationThetaOffsetUnits=deg  RotationMethod=ArbitraryAxis  RotationAngleUnits=rad  RotationStandardAxis=+Z  RotationAngle=1.624664356272121  RotationArbitraryAxis=[-0.22603347840136134 0.22603347840136132 0.94753244444903439]  FollAlignAxisA=+X  BaseAlignAxisA=+Y  FollAlignAxisB=+Y  BaseAlignAxisB=+Z  RotationSequenceAxes=FollowerAxes  RotationSequence=XYX  RotationSequenceAngles=[0 0 0]  RotationSequenceAnglesUnits=deg  RotationMatrix=[1 0 0; 0 1 0; 0 0 1]
  F : PMIOPort  Side=Left
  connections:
  Transform/LConn1 -- ReferenceFrame/RConn1 -- Transform1/LConn1 -- Transform2/LConn1
  Transform/RConn1 -- F/RConn1
  ROTOR_1_RIGID/LConn1 -- Transform1/RConn1
  CODEUR_1_RIGID/LConn1 -- Transform2/RConn1
